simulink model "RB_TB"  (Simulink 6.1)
settings: Solver=ode3  SolverMode=SingleTasking  StartTime=0  StopTime=1000  FixedStep=0.05  RelTol=1e-3
libraries: simulink x2
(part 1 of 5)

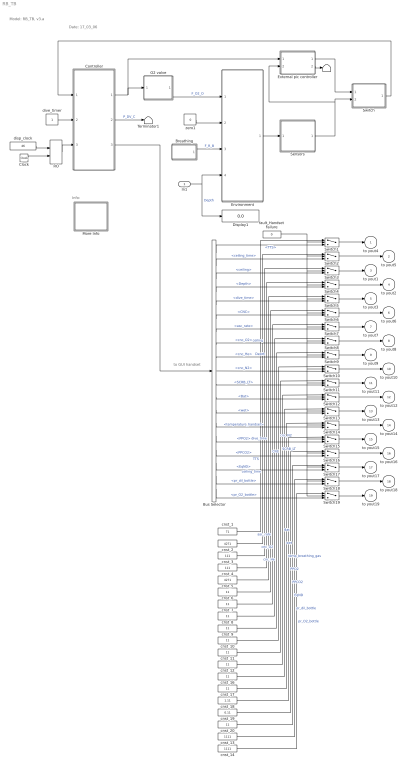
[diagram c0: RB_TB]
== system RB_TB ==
  note: Model: RB_TB, v3.a
  note: Date: 17_03_06
  note: to GUI handset
  note: Info:
  In1 : Inport  Port=1  LatchInput=off
  Breathing : Subsystem
  Bus Selector : BusSelector  DialogController=Simulink.DDGSource_Bus  OutputSignals=TTS,ceiling_time,ceiling,Depth,dive_time,CNC,asc_rate,cnc_O2,cnc_He,cnc_N2,SCRB_LT,Bat,wet,temperature_handset,PPO2,PPCO2,EqND,pr_dil_bottle,pr_O2_bottle
  Clock : Clock
  Controller : Subsystem
  Display1 : Display
  Environment : Subsystem
  External pic controller : Subsystem
  More Info : Subsystem
  O2 valve : Subsystem
  RO : RelationalOperator  Operator===  LogicOutDataTypeMode=Boolean
  Sensors : Subsystem
  Switch : Subsystem
  Switch{1..19} (19 alike) : Switch  Threshold=0.5
  T : Terminator
  Terminator1 : Terminator
  cnst_1 : Constant  Value=71
  cnst_{6..12,16..17,20} (10 alike) : Constant  Value=11
  cnst_13 : Constant  Value=1111
  cnst_14 : Constant  Value=1111
  cnst_18 : Constant  Value=1.11
  cnst_19 : Constant  Value=0.11
  cnst_2 : Constant  Value=4271
  cnst_3 : Constant  Value=111
  cnst_4 : Constant  Value=111
  cnst_5 : Constant  Value=4271
  disp_clock : Constant  Value=46
  dive_timer : Constant
  fault_Handset Failure : Constant  Value=0
  zero1 : Constant  Value=0
  to yout4 : Outport
  to yout5 : Outport  Port=2
  to yout1 : Outport  Port=3
  to yout2 : Outport  Port=4
  to yout3 : Outport  Port=5
  to yout6 : Outport  Port=6
  to yout7 : Outport  Port=7
  to yout8 : Outport  Port=8
  to yout9 : Outport  Port=9
  to yout10 : Outport  Port=10
  to yout11 : Outport  Port=11
  to yout12 : Outport  Port=12
  to yout13 : Outport  Port=13
  to yout14 : Outport  Port=14
  to yout15 : Outport  Port=15
  to yout16 : Outport  Port=16
  to yout17 : Outport  Port=17
  to yout18 : Outport  Port=18
  to yout19 : Outport  Port=19
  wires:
  Controller/1(O2 control) -> O2 valve/1(IN), External pic controller/1(valve_in)
  Breathing/1(Metabolic) -> Environment/3(Metablic)  "F_R_B"
  Environment/1(bus) -> Sensors/1(In)
  disp_clock/1 -> RO/1
  Clock/1 -> RO/2
  RO/1 -> Controller/3(disp_clock)
  External pic controller/1(sensor_out) -> Switch/1(In1)
  Sensors/1(Out) -> Switch/2(In2), External pic controller/2(sensor_in)
  Switch/1(Out) -> Controller/1(InBus)
  Controller/2(Dil valve) -> Terminator1/1  "P_DV_C"
  zero1/1 -> Environment/2(Dil valve)
  O2 valve/1(Orf_size) -> Environment/1(Orf_size)  "F_O2_O"
  dive_timer/1 -> Controller/2(dive_timer)
  cnst_1/1 -> Switch1/1  "TTS"
  cnst_2/1 -> Switch2/1  "ceiling_time"
  cnst_3/1 -> Switch3/1  "ceiling"
  cnst_4/1 -> Switch4/1  "Depth"
  cnst_5/1 -> Switch5/1  "dive_time"
  cnst_6/1 -> Switch6/1  "CNC"
  cnst_7/1 -> Switch7/1  "asc_rate"
  cnst_8/1 -> Switch8/1  "cnc_O2"
  cnst_9/1 -> Switch9/1  "cnc_He"
  cnst_10/1 -> Switch10/1  "cnc_N2"
  cnst_11/1 -> Switch11/1  "SCRB_LT"
  cnst_12/1 -> Switch12/1  "Bat"
  cnst_16/1 -> Switch13/1  "wet"
  cnst_17/1 -> Switch14/1  "temp_breathing_gas"
  cnst_18/1 -> Switch15/1  "PPO2"
  cnst_19/1 -> Switch16/1  "PPCO2"
  cnst_20/1 -> Switch17/1  "EqND"
  cnst_13/1 -> Switch18/1  "pr_dil_bottle"
  cnst_14/1 -> Switch19/1  "pr_O2_bottle"
  Controller/3(bus) -> Bus Selector/1
  Bus Selector/1 -> Switch1/3  "<TTS>"
  Bus Selector/2 -> Switch2/3  "<ceiling_time>"
  Bus Selector/3 -> Switch3/3  "<ceiling>"
  Bus Selector/4 -> Switch4/3  "<Depth>"
  Bus Selector/5 -> Switch5/3  "<dive_time>"
  Bus Selector/6 -> Switch6/3  "<CNC>"
  Bus Selector/7 -> Switch7/3  "<asc_rate>"
  Bus Selector/8 -> Switch8/3  "<cnc_O2>"
  Bus Selector/9 -> Switch9/3  "<cnc_He>"
  Bus Selector/10 -> Switch10/3  "<cnc_N2>"
  Bus Selector/11 -> Switch11/3  "<SCRB_LT>"
  Bus Selector/12 -> Switch12/3  "<Bat>"
  Bus Selector/13 -> Switch13/3  "<wet>"
  Bus Selector/14 -> Switch14/3  "<temperature_handset>"
  Bus Selector/15 -> Switch15/3  "<PPO2>"
  Bus Selector/16 -> Switch16/3  "<PPCO2>"
  Bus Selector/17 -> Switch17/3  "<EqND>"
  Bus Selector/18 -> Switch18/3  "<pr_dil_bottle>"
  Bus Selector/19 -> Switch19/3  "<pr_O2_bottle>"
  Switch19/1 -> to yout19/1
  Switch18/1 -> to yout18/1
  Switch17/1 -> to yout17/1
  Switch16/1 -> to yout16/1
  Switch15/1 -> to yout15/1
  Switch14/1 -> to yout14/1
  Switch13/1 -> to yout13/1
  Switch12/1 -> to yout12/1
  Switch11/1 -> to yout11/1
  Switch10/1 -> to yout10/1
  Switch9/1 -> to yout9/1
  Switch8/1 -> to yout8/1
  Switch7/1 -> to yout7/1
  Switch6/1 -> to yout6/1
  Switch5/1 -> to yout3/1
  Switch4/1 -> to yout2/1
  Switch3/1 -> to yout1/1
  Switch2/1 -> to yout5/1
  Switch1/1 -> to yout4/1
  fault_Handset Failure/1 -> Switch18/2, Switch19/2, Switch17/2, Switch16/2, Switch15/2, Switch14/2, Switch13/2, Switch12/2, Switch11/2, Switch10/2, Switch9/2, Switch8/2, Switch7/2, Switch6/2, Switch5/2, Switch4/2, Switch3/2, Switch2/2, Switch1/2
  In1/1 -> Display1/1, Environment/4(Depth)  "Depth"
  External pic controller/2(valve_out) -> T/1

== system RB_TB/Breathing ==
  note: Model: RB_TB/Breathing
  methabolic profile 1l/s : DiscretePulseGenerator  PulseType=Time based  Amplitude=2.5  PulseWidth=40
  product1 : Product
  rate_metabolic : Constant  Value=1.88
  scale : Gain  Gain=1/60
  Metabolic : Outport
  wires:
  methabolic profile 1l/s/1 -> product1/2
  product1/1 -> Metabolic/1  "l/s"
  scale/1 -> product1/1  "l/s"
  rate_metabolic/1 -> scale/1  "l/min"

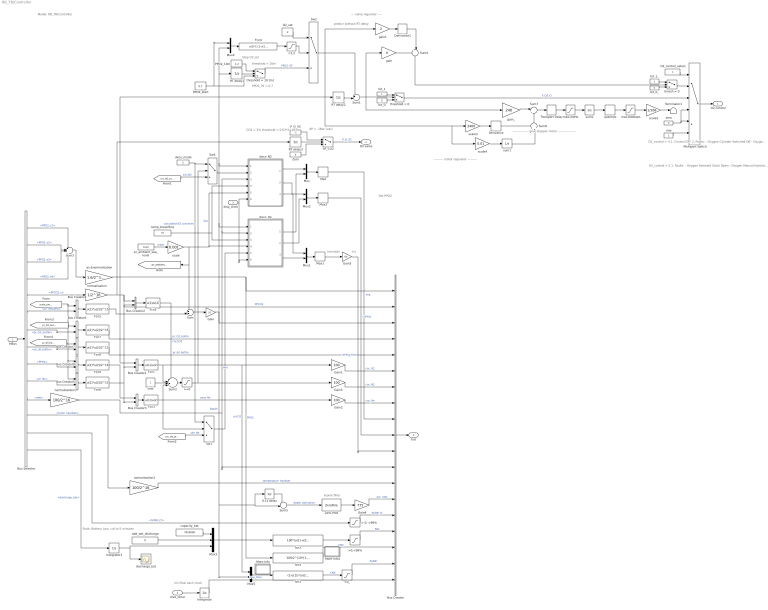
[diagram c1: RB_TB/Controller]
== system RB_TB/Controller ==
  note: Model: RB_TB/Controller
  note: dP = -1Bar (var)
  note: PPO2_ini = 0.7
  note: threshold = 10m
  note: CO2 = 3% threshold = 0.03*2^16
  note: (minute)
  note: (s)
  note: Step O2 set
  note: ini=final each clock
  note: Fault: Battery Low, cut to 5 minutes
  note: predicr without RT delay
  note: O2_control = 4 1. Control OFF 2. Faults: - Oxygen Cylinder Switched Off - Oxygen First Stage Failure - Oxygen Solenoid Stuck Closed
  note: O2_control = 5 1. Faults: - Oxygen Solenoid Stuck Open - Oxygen Manual Injector Failure
  note: 6-pole filter
  note: --------------- gear stepper motor -----------------
  note: Set PPO2
  note: --------- motor regulator ---------
  note: --- valve regulator ----
  InBus : Inport  Port=1  LatchInput=off
  dive_timer : Inport  Port=2  LatchInput=off
  disp_clock : Inport  Port=3  LatchInput=off
  0.1s delay : UnitDelay  SampleTime=0.1
  <1.2 : Saturate  UpperLimit=1.2  LowerLimit=0
  "> 0, <99%" : Saturate  UpperLimit=99  LowerLimit=0
  >0,<99% : Saturate  UpperLimit=99  LowerLimit=0
  >0_ : Saturate  UpperLimit=inf  LowerLimit=0
  >=0 : Saturate  UpperLimit=inf  LowerLimit=0
  Bus Creator : BusCreator  DialogController=Simulink.DDGSource_Bus  Inputs=19
  Bus Creator{1..8} (8 alike) : BusCreator  DialogController=Simulink.DDGSource_Bus  Inputs=2
  Bus Selector : BusSelector  DialogController=Simulink.DDGSource_Bus  OutputSignals=PPO2_s1,PPO2_s2,PPO2_s3,PPO2_s4,PPCO2_s,pr_ambient,pr_O2_bottle,pr_dil_bottle,PPHe,pr_BL,wet,temp_handset,SCRB_LT,discharge_bat
  Derivative : Derivative
  Derivative1 : Derivative
  Fcn1 : Fcn  Expr=u(1)/u(2)
  Fcn2 : Fcn  Expr=u(1)/u(2)
  Fcn3 : Fcn  Expr=u(1)/u(2)
  Fcn4 : Fcn  Expr=u(2)*(1.2-u(1))/10+u(1)
  Fcn{5..8} (4 alike) : Fcn  Expr=u(1)*u(2)/2^15
  Fcn9 : Fcn  Expr=u(1)*u(2)/2^16
  Gain : Gain  Gain=10
  Gain1 : Gain  Gain=100
  Gain2 : Gain  Gain=100
  Gain3 : Gain  Gain=60
  Gain4 : Gain  Gain=775
  Gain5 : Gain  Gain=100
  Integrator : Integrator
  Integrator1 : Integrator
  Max : MinMax  Function=max
  Max1 : MinMax  Function=max
  Max2 : MinMax  Function=max
  More Info : Subsystem
  More Info1 : Subsystem
  Multiport Switch : MultiPortSwitch  Inputs=5
  Mux{,1..2,4..5} (5 alike) : Mux  Inputs=2
  Mux3 : Mux  Inputs=3
  O2_control_select : Constant
  O2_set : Constant  Value=2
  PPO2_10m : Constant  Value=1.2
  PPO2_start : Constant  Value=0.7
  P_D_VC : Constant  Value=-1
  RT delay1 : UnitDelay  SampleTime=0.1
  RT delay2 : UnitDelay  SampleTime=0.1
  RT delay3 : UnitDelay  SampleTime=0.1
  SP_CO2 : Switch  Threshold=0.03
  Sum : Sum  Inputs=-+|
  Sum1 : Sum  Inputs=+-|
  Sum2 : Sum  Inputs=--+-|
  Sum3 : Sum  Inputs=++++
  Sum4 : Sum  Orientation=down  Inputs=+-|
  Sum5 : Sum  Inputs=-+|
  Sum7 : Sum  Inputs=|+-
  Sum8 : Sum  Orientation=up  Inputs=++|
  Sw1 : MultiPortSwitch  Inputs=2
  Sw2 : MultiPortSwitch  Inputs=2
  Sw4 : MultiPortSwitch  Inputs=2
  Terminator1 : Terminator
  Transport Delay : TransportDelay  DelayTime=0.01
  Zero : Constant  Value=0
  Zero-Pole : ZeroPole  Zeros=[0]  Poles=[-1 -1 -1 -1 -1 -1]
  add_bat_discharge : Constant  Value=0
  av.&normalisation : Gain  Gain=1.6/2^16/4
  bit_0 : Constant  Value=0
  bit_0_ : Constant  Value=0
  bit_1 : Constant
  bit_1_ : Constant
  capacity_bat : Constant  Value=7920000
  cnst : Constant
  deco_He : Subsystem
  deco_N2 : Subsystem
  deco_mode : Constant  Value=2
  discharge_bat : Scope
  fcn2 : Fcn  Expr=100*(u(1)-u(2)-u(3))/u(1)
  fcn3 : Fcn  Expr=(1-u(1))*(u(2)+10)/0.79-10
  fcn4 : Fcn  Expr=100/2^(10*(1.6 - u(1)))
  gain : Gain
  gain1 : Gain  Gain=2
  gain_ : Gain  Gain=240
  max100Hz : Saturate  UpperLimit=100  LowerLimit=-100
  max168steps : Saturate  UpperLimit=168  LowerLimit=0
  normalisation : Gain  Gain=1/2^16
  normalisation1 : Gain  Gain=100/2^16
  normalisation2 : Gain  Gain=100/2^16
  one : Constant
  pr_ambient_sea_level : Constant  Value=1010
  quantize : Quantizer  QuantizationInterval=1
  scale : Gain  Gain=0.001
  scale2 : Gain  Gain=1/168
  scale3 : Gain  Gain=3400
  scale4 : Gain  Gain=0.01
  sum1 : Integrator
  sum2 : Integrator
  temp_breathing : Constant  Value=33
  thresh = 0 : Switch  Criteria=u2 > Threshold
  threshold = 0 : Switch  Criteria=u2 > Threshold
  threshold = 10 [m] : Switch  Threshold=10
  zero : Constant  Value=0
  O2 control : Outport
  Dil valve : Outport  Port=2
  bus : Outport  Port=3
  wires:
  RT delay2/1 -> Sum1/2
  RT delay1/1 -> threshold = 10 [m]/2
  PPO2_start/1 -> threshold = 10 [m]/3, Mux4/1
  PPO2_10m/1 -> threshold = 10 [m]/1
  bit_1/1 -> threshold = 0/1
  bit_0/1 -> threshold = 0/3
  temp_breathing/1 -> deco_N2/4(Temp_air), deco_He/3(Temp_air)
  deco_N2/1(TTS_N2) -> Mux/1
  deco_He/1(TTS_He) -> Mux/2
  Mux/1 -> Max/1
  Mux1/1 -> Max1/1
  deco_He/3(ceiling_time_He) -> Mux1/2
  deco_N2/3(ceiling_time_N2) -> Mux1/1
  Mux2/1 -> Max2/1
  deco_N2/2(ceiling_N2) -> Mux2/1
  deco_He/2(ceiling_He) -> Mux2/2
  Max/1 -> Bus Creator/9  "TTS"
  Max2/1 -> Bus Creator/10  "ceiling"
  pr_ambient_sea_level/1 -> scale/1  "mbar"
  Bus Creator/1 -> bus/1
  InBus/1 -> Bus Selector/1
  Bus Selector/3 -> Sum3/3  "<PPO2_s3>"
  Bus Selector/4 -> Sum3/4  "<PPO2_s4>"
  av.&normalisation/1 -> Bus Creator1/1, Bus Creator/1, fcn4/1, RT delay2/1, gain1/1, scale3/1, scale4/1  "PPO2"
  normalisation/1 -> RT delay3/1, Bus Creator2/1, Bus Creator/2  "PPCO2"
  Sum/1 -> Gain/1
  Gain/1 -> Bus Creator/3, deco_He/1(depth), deco_N2/1(depth), RT delay1/1, Mux4/2, Mux5/2, 0.1s delay/1, Sum5/2  "Depth"
  Gain5/1 -> Bus Creator/7  "cnc_N2"
  Fcn3/1 -> Sum2/4, Sw1/2, Gain2/1  "sens He"
  disp_clock/1 -> deco_N2/6(disp_clock), deco_He/6(disp_clock)
  Integrator/1 -> Bus Creator/19  "dive_time"
  >0,<99%/1 -> Bus Creator/16  "Bat"
  >0_/1 -> Bus Creator/18  "EqND"
  RT delay3/1 -> SP_CO2/2
  P_D_VC/1 -> SP_CO2/1
  SP_CO2/1 -> Dil valve/1  "P_D_VC"
  Zero/1 -> SP_CO2/3
  Bus Selector/5 -> normalisation/1  "<PPCO2_s>"
  scale/1 -> deco_He/4(P_amb_sea_level), deco_N2/5(P_amb_sea_level), Sum/1, [pr_ambient_sea_level]  "bar"
  Max1/1 -> Gain3/1
  Gain3/1 -> Bus Creator/11  "ceiling_time"
  Mux3/1 -> fcn2/1
  fcn2/1 -> >0,<99%/1
  Fcn1/1 -> Sum2/2, Gain1/1, Mux5/1  "cncO2"
  Gain1/1 -> Bus Creator/6  "cnc_O2"
  Gain2/1 -> Bus Creator/8  "cnc_He"
  Bus Creator2/1 -> Fcn2/1
  cnst/1 -> Sum2/3
  Fcn2/1 -> Sum2/1  "cncCO2"
  deco_mode/1 -> Sw4/1, Sw1/1
  [cnc_N2_presize] -> Sw4/3  "sim N2"
  [cnc_He_presize] -> Sw1/3  "sim He"
  Sw4/1 -> deco_N2/2(cnc_N2)
  Sw1/1 -> deco_He/5(cnc_He)
  O2_set/1 -> Sw2/1
  threshold = 10 [m]/1 -> Sw2/3  "PPO2_SP"
  Sw2/1 -> Sum1/1
  Mux4/1 -> Fcn4/1
  <1.2/1 -> Sw2/2
  Fcn4/1 -> <1.2/1
  Mux5/1 -> fcn3/1
  fcn3/1 -> >0_/1  "CNS"
  fcn4/1 -> Bus Creator/17  "CNC"
  dive_timer/1 -> Integrator/1
  capacity_bat/1 -> Mux3/1
  add_bat_discharge/1 -> Mux3/2
  Integrator1/1 -> discharge_bat/1, Mux3/3
  Bus Selector/2 -> Sum3/2  "<PPO2_s2>"
  Bus Selector/1 -> Sum3/1  "<PPO2_s1>"
  Sum3/1 -> av.&normalisation/1
  Sum1/1 -> gain/1, threshold = 0/2, gain_/1
  gain1/1 -> Derivative1/1
  O2_control_select/1 -> Multiport Switch/1
  Multiport Switch/1 -> O2 control/1
  bit_1_/1 -> thresh = 0/1
  bit_0_/1 -> thresh = 0/3
  Sum4/1 -> thresh = 0/2
  thresh = 0/1 -> Multiport Switch/2
  threshold = 0/1 -> Multiport Switch/3  "F_O2_O"
  "> 0, <99%"/1 -> Bus Creator/15  "SCRB_LT"
  Bus Selector/14 -> Integrator1/1  "<discharge_bat>"
  Bus Selector/13 -> "> 0, <99%"/1  "<SCRB_LT>"
  Bus Selector/11 -> normalisation1/1  "<wet>"
  normalisation1/1 -> deco_He/2(Wet), deco_N2/3(Wet), Bus Creator/12  "wet"
  Bus Selector/12 -> normalisation2/1  "<temp_handset>"
  normalisation2/1 -> Bus Creator/13  "temperature_handset"
  [scale_pressure] -> Bus Creator4/1, Bus Creator5/1, Bus Creator8/1
  Bus Selector/6 -> Bus Creator4/2  "<pr_ambient>"
  Bus Creator4/1 -> Fcn5/1
  Fcn5/1 -> Sum/2
  Sum2/1 -> >=0/1
  >=0/1 -> Gain5/1, Sw4/2  "calculated N2 concentration"
  one/1 -> Multiport Switch/6
  zero/1 -> Multiport Switch/5, Multiport Switch/4
  Bus Creator3/1 -> Fcn3/1
  Bus Creator1/1 -> Fcn1/1
  Bus Creator5/1 -> Fcn6/1
  Bus Selector/10 -> Bus Creator5/2  "<pr_BL>"
  Fcn6/1 -> Bus Creator3/2, Bus Creator1/2, Bus Creator2/2
  Sum5/1 -> Zero-Pole/1  "depth_derivative"
  0.1s delay/1 -> Sum5/1
  Zero-Pole/1 -> Gain4/1
  Gain4/1 -> Bus Creator/14  "asc_rate"
  Bus Selector/7 -> Bus Creator6/2  "<pr_O2_bottle>"
  Fcn7/1 -> Bus Creator/4  "pr_O2_bottle"
  Bus Creator6/1 -> Fcn7/1
  [pr_O2_bottle_ini] -> Bus Creator6/1
  Bus Creator7/1 -> Fcn8/1
  Fcn8/1 -> Bus Creator/5  "pr_dil_bottle"
  Bus Selector/8 -> Bus Creator7/2  "<pr_dil_bottle>"
  [pr_dil_bottle_ini] -> Bus Creator7/1
  Bus Creator8/1 -> Fcn9/1
  Bus Selector/9 -> Bus Creator8/2  "<PPHe>"
  Fcn9/1 -> Bus Creator3/1
  max168steps/1 -> scale2/1
  quantize/1 -> max168steps/1
  sum2/1 -> quantize/1
  max100Hz/1 -> sum2/1
  Transport Delay/1 -> max100Hz/1
  Sum7/1 -> Transport Delay/1
  scale3/1 -> Derivative/1
  scale4/1 -> sum1/1
  gain_/1 -> Sum7/1
  Derivative/1 -> Sum8/1
  Sum8/1 -> Sum7/2
  gain/1 -> Sum4/1
  Derivative1/1 -> Sum4/2
  sum1/1 -> Sum8/2
  scale2/1 -> Terminator1/1

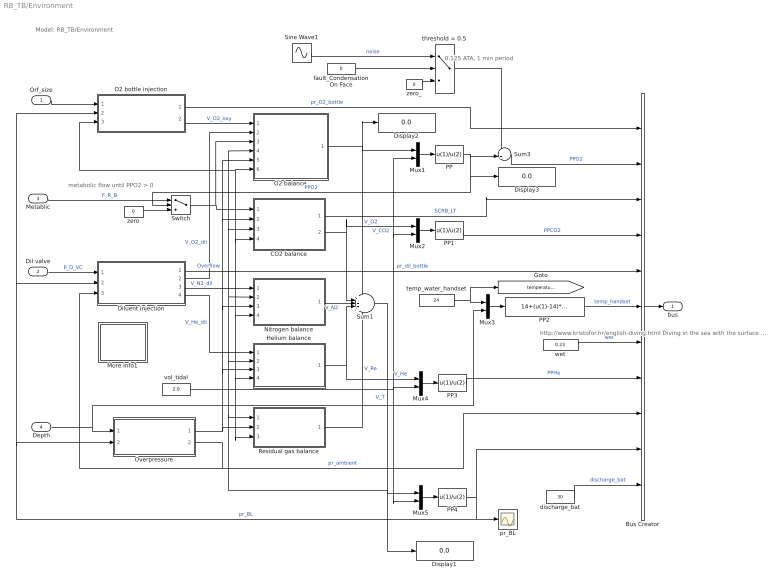
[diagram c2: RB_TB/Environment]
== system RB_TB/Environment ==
  note: Model: RB_TB/Environment
  note: metabolic flow until PPO2 > 0
  note: 0.125 ATA, 1 min period
  note: http://www.kristofor.hr/english-diving.html Diving in the sea with the surface sea temperature 9 - 12 deg.C in winter, 24 - 28 degC in summer, On 20 m sea depth temperature is permanent, around 14 deg.C
  Orf_size : Inport  Port=1  LatchInput=off
  Dil valve : Inport  Port=2  LatchInput=off
  Metablic : Inport  Port=3  LatchInput=off
  Depth : Inport  Port=4  LatchInput=off
  Bus Creator : BusCreator  DialogController=Simulink.DDGSource_Bus  Inputs=11
  CO2 balance : Subsystem
  Diluent injection : Subsystem
  Display1 : Display
  Display2 : Display
  Display3 : Display
  Helium balance : Subsystem
  More Info1 : Subsystem
  Mux{1..5} (5 alike) : Mux  Inputs=2
  Nitrogen balance : Subsystem
  O2 balance : Subsystem
  O2 bottle injection : Subsystem
  Overpressure : Subsystem
  PP{,1,3..4} (4 alike) : Fcn  Tag=ee  Priority=306454640  Expr=u(1)/u(2)
  PP2 : Fcn  Tag=ee  Priority=306454640  Expr=14+(u(1)-14)*exp(-u(2)/7)
  Residual gas balance : Subsystem
  Sine Wave1 : Sin  Amplitude=0.125  Frequency=pi/30  SampleTime=0
  Sum1 : Sum  Inputs=+++++
  Sum3 : Sum  Inputs=++|
  Switch : Switch  Criteria=u2 > Threshold
  discharge_bat : Constant  Value=30
  fault_Condensation On Face : Constant  Value=0
  pr_BL : Scope
  temp_water_handset : Constant  Value=24
  threshold = 0.5 : Switch  Criteria=u2 > Threshold  Threshold=0.5
  vol_tidal : Constant  Value=2.0
  wet : Constant  Value=0.23
  zero : Constant  Value=0
  zero_ : Constant  Value=0
  bus : Outport
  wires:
  Diluent injection/3(N2) -> Nitrogen balance/1(V_N2_dil)  "V_N2_dil"
  Diluent injection/2(O2) -> O2 balance/2(V_O2_dil)  "V_O2_dil"
  O2 balance/1(O2 inside) -> Sum1/1, Mux1/1, Display2/1  "V_O2"
  Overpressure/1(Overflow) -> CO2 balance/2(Overflow), O2 balance/5(Overflow), Nitrogen balance/3(Overflow), Helium balance/3(Overflow), Residual gas balance/2(Overflow)  "Overflow"
  Sum1/1 -> Mux5/1, Helium balance/2(gas_total), Nitrogen balance/2(gas_total), CO2 balance/3(gas_total), O2 balance/4(gas_total), Residual gas balance/1(gas_total), Display1/1  "V_T"
  Nitrogen balance/1(N2 inside) -> Sum1/3  "V_N2"
  CO2 balance/2(CO2) -> Sum1/2, Mux2/1  "V_CO2"
  Dil valve/1 -> Diluent injection/1(Valve_ON/OFF)  "P_D_VC"
  Helium balance/1(He inside) -> Mux4/1, Sum1/4  "V_He"
  Diluent injection/4(He) -> Helium balance/1(V_He_dil)  "V_He_dil"
  Residual gas balance/1(Re inside) -> Sum1/5  "V_Re"
  PP/1 -> Sum3/2, Switch/2, Display3/1  "PPO2"
  Bus Creator/1 -> bus/1
  PP1/1 -> Bus Creator/4  "PPCO2"
  PP3/1 -> Bus Creator/8  "PPHe"
  vol_tidal/1 -> Helium balance/4(vol_tidal), Nitrogen balance/4(vol_tidal), CO2 balance/4(vol_tidal), O2 balance/6(vol_tidal), O2 bottle injection/3(vol_tidal), Residual gas balance/3(vol_tidal), Mux4/2, Mux2/2, Mux1/2, Mux5/2
  Mux1/1 -> PP/1
  Mux2/1 -> PP1/1
  Mux4/1 -> PP3/1
  Orf_size/1 -> O2 bottle injection/1(Orf_size)
  O2 bottle injection/2(V_O2_oxygen_bottle) -> O2 balance/1(V_O2_oxy)  "V_O2_oxy"
  O2 bottle injection/1(pr_O2_bottle) -> Bus Creator/1  "pr_O2_bottle"
  wet/1 -> Bus Creator/7  "wet"
  Overpressure/2(pr_ambient) -> Bus Creator/9, Diluent injection/3(pr_ambient)  "pr_ambient"
  Diluent injection/1(pr_dil_bottle) -> Bus Creator/5  "pr_dil_bottle"
  Mux5/1 -> PP4/1
  PP4/1 -> Bus Creator/10, pr_BL/1, O2 bottle injection/2(pr_BL), Diluent injection/2(pr_BL), Overpressure/2(pr_BL)  "pr_BL"
  Depth/1 -> Overpressure/1(Depth), Mux3/2
  Switch/1 -> CO2 balance/1(Metabolic), O2 balance/3(Metabolic)
  Metablic/1 -> Switch/1  "F_R_B"
  zero/1 -> Switch/3
  CO2 balance/1(SCRB) -> Bus Creator/3  "SCRB_LT"
  discharge_bat/1 -> Bus Creator/11  "discharge_bat"
  fault_Condensation On Face/1 -> threshold = 0.5/2
  Sine Wave1/1 -> threshold = 0.5/1  "noise"
  zero_/1 -> threshold = 0.5/3
  Sum3/1 -> Bus Creator/2  "PPO2"
  threshold = 0.5/1 -> Sum3/1
  temp_water_handset/1 -> Mux3/1, [temperature_sea_level]
  Mux3/1 -> PP2/1
  PP2/1 -> Bus Creator/6  "temp_handset"

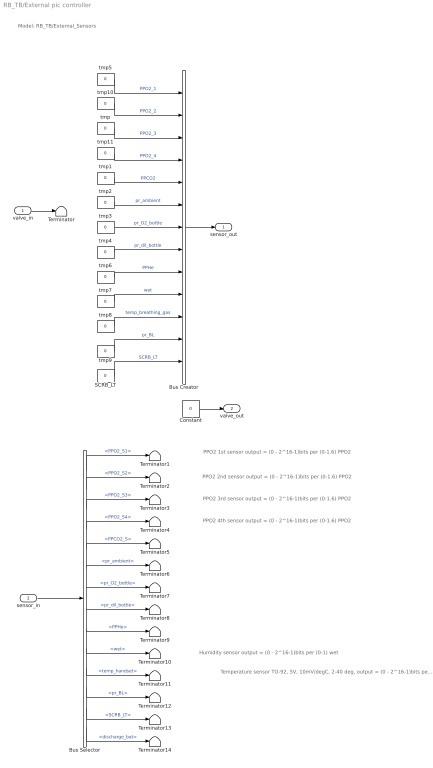
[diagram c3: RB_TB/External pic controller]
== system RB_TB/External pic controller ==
  note: Model: RB_TB/External_Sensors
  note: Humidity sensor output = (0 - 2^16-1)bits per (0-1) wet
  note: PPO2 1st sensor output = (0 - 2^16-1)bits per (0-1.6) PPO2
  note: PPO2 2nd sensor output = (0 - 2^16-1)bits per (0-1.6) PPO2
  note: PPO2 3rd sensor output = (0 - 2^16-1)bits per (0-1.6) PPO2
  note: PPO2 4th sensor output = (0 - 2^16-1)bits per (0-1.6) PPO2
  note: Temperature sensor TO-92, 5V, 10mV/degC, 2-40 deg, output = (0 - 2^16-1)bits per (0-1) wet
  valve_in : Inport  Port=1  LatchInput=off
  sensor_in : Inport  Port=2  LatchInput=off
  Bus Creator : BusCreator  DialogController=Simulink.DDGSource_Bus  Inputs=13
  Bus Selector : BusSelector  DialogController=Simulink.DDGSource_Bus  OutputSignals=PPO2_S1,PPO2_S2,PPO2_S3,PPO2_S4,PPCO2_S,pr_ambient,pr_O2_bottle,pr_dil_bottle,PPHe,wet,temp_handset,pr_BL,SCRB_LT,discharge_bat
  Constant : Constant  Value=0
  SCRB_LT : Constant  Value=0
  Terminator{,1..14} (15 alike) : Terminator
  tmp{,1..11} (12 alike) : Constant  Value=0
  sensor_out : Outport
  valve_out : Outport  Port=2
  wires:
  tmp7/1 -> Bus Creator/10  "wet"
  tmp8/1 -> Bus Creator/11  "temp_breathing_gas"
  tmp6/1 -> Bus Creator/9  "PPHe"
  tmp4/1 -> Bus Creator/8  "pr_dil_bottle"
  tmp3/1 -> Bus Creator/7  "pr_O2_bottle"
  tmp2/1 -> Bus Creator/6  "pr_ambient"
  tmp1/1 -> Bus Creator/5  "PPCO2"
  Bus Creator/1 -> sensor_out/1
  tmp/1 -> Bus Creator/3  "PPO2_3"
  valve_in/1 -> Terminator/1
  tmp9/1 -> Bus Creator/12  "pr_BL"
  SCRB_LT/1 -> Bus Creator/13  "SCRB_LT"
  tmp5/1 -> Bus Creator/1  "PPO2_1"
  tmp10/1 -> Bus Creator/2  "PPO2_2"
  sensor_in/1 -> Bus Selector/1
  tmp11/1 -> Bus Creator/4  "PPO2_4"
  Bus Selector/1 -> Terminator1/1  "<PPO2_S1>"
  Bus Selector/2 -> Terminator2/1  "<PPO2_S2>"
  Bus Selector/3 -> Terminator3/1  "<PPO2_S3>"
  Bus Selector/4 -> Terminator4/1  "<PPO2_S4>"
  Bus Selector/5 -> Terminator5/1  "<PPCO2_S>"
  Bus Selector/9 -> Terminator9/1  "<PPHe>"
  Bus Selector/6 -> Terminator6/1  "<pr_ambient>"
  Bus Selector/7 -> Terminator7/1  "<pr_O2_bottle>"
  Bus Selector/8 -> Terminator8/1  "<pr_dil_bottle>"
  Bus Selector/10 -> Terminator10/1  "<wet>"
  Bus Selector/11 -> Terminator11/1  "<temp_handset>"
  Bus Selector/12 -> Terminator12/1  "<pr_BL>"
  Bus Selector/13 -> Terminator13/1  "<SCRB_LT>"
  Bus Selector/14 -> Terminator14/1  "<discharge_bat>"
  Constant/1 -> valve_out/1

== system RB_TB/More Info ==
  note: The S-Function "depth_data" runs depth_data.m in real-time that calculates the current depth using the Depth table data. The Simulink subsytems are Valve controller and Breathing loop. Gas balance includes O2, CO2, N2, He and Reminder gas the O2 pressure reduction valve is not compensated to ambient pressure Controller includes: Bang-Bang O2 and CO2 control; calc of decompression The depth profile is profile.time = [time1, time2,..., timen], and profile.rate = [depth_ini, rate1, rate2,...raten ] 1b deco compartments for N2 and He are installed "a", "b" and Half-Time deco for H2 is updated tissue compartment of 1b deco for N2 and He are add the half_times of He are updated satuation of the PPO2 sensor is 1.6 round of the deco d_min is changed by ceil ceil of the deco ceiling time and asc_time is removed models of the SCRB, BAT, CNS and EqND parameters are installed 04_03_06 updated (limit is -inf) the non compensated O2 valve 05_03_06 compensated O2 valve is installed 08_03_06 flow through the orifice depends on its diameter and spring pressure 08_03_06 ADV and OVP value of 5-50mbar is defined via the GUI 09_03_06 Faults are attached 11_03_06 Range of Analog O2 set is (0.7 - 1.2 ATA)/(0-10m) 18_03_06 Nonlinear model of OPV and ADV valves are installed 18_03_06 Predictive Bang-Bang O2 valve control is installed 22_03_06 PPO2 and CO2 LED are installed 23_03_06 Sensors time constant and ADCs are installed 24_03_06 O2 and Dil manual injection is add 25_03_06 Sound of PAUSE and nonconnected modes is ON
  note: The run file is main_RB_TB.m
  note: Temporary actions: 1) The 0.1s delay of PPO2 sensor is removed
  note: This system models the Re-Breather Test Bench. It includs analogue and digital parts.
  note: PPCO2 controls is off

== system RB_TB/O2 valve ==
  note: Model: RB_TB/O2 valve
  IN : Inport  Port=1  LatchInput=off
  DAC 1bit : DataTypeConversion  OutDataTypeMode=double  ConvertRealWorld=Stored Integer (SI)  RndMeth=Nearest
  Orf_size : Outport
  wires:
  IN/1 -> DAC 1bit/1
  DAC 1bit/1 -> Orf_size/1

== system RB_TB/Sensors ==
  note: Model: RB_TB/Sensors
  note: Info:
  note: 5 mV corresponds to air PPO2 of 0.21 ATA
  In : Inport  Port=1  LatchInput=off
  5mV : Constant  Value=8580.1
  Bus Creator : BusCreator  DialogController=Simulink.DDGSource_Bus  Inputs=14
  Bus Selector : BusSelector  DialogController=Simulink.DDGSource_Bus  OutputSignals=PPO2,PPCO2,pr_ambient,pr_O2_bottle,pr_dil_bottle,PPHe,wet,temp_handset,pr_BL,SCRB_LT,discharge_bat
  Gain : Gain
  Gain1 : Gain
  Gain2 : Gain
  Humidity Sensor : Subsystem
  More Info : Subsystem
  PPCO2 sensor : Subsystem
  PPHe sensor : Subsystem
  PPO2 sensor : Subsystem
  Pressure_Br_Loop Sensor : Subsystem
  Pressure_O2_bottle_Sensor1 : Subsystem
  Pressure_ambient Sensor : Subsystem
  Pressure_dil_bottle_Sensor : Subsystem
  Temperature Sensor : Subsystem
  fault_Loose Connection to Sensor : Constant  Value=0
  fault_Single Cell Failure : Constant  Value=0
  fault_Two Cell Failure : Constant  Value=0
  thresh = 0.5 : Switch  Criteria=u2 > Threshold  Threshold=0.5
  threshold = 0.5 : Switch  Criteria=u2 > Threshold  Threshold=0.5
  threshold = 0.5_ : Switch  Criteria=u2 > Threshold  Threshold=0.5
  zero : Constant  Value=0
  Out : Outport
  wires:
  In/1 -> Bus Selector/1
  Bus Creator/1 -> Out/1
  Bus Selector/1 -> PPO2 sensor/1(PPO2)  "<PPO2>"
  Bus Selector/2 -> PPCO2 sensor/1(PPCO2)  "<PPCO2>"
  PPO2 sensor/1(PPO2_S) -> threshold = 0.5/3  "PPO2_S"
  PPCO2 sensor/1(PPCO2_S) -> Bus Creator/5  "PPCO2_S"
  Bus Selector/10 -> Bus Creator/13  "<SCRB_LT>"
  Bus Selector/11 -> Bus Creator/14  "<discharge_bat>"
  fault_Loose Connection to Sensor/1 -> threshold = 0.5/2
  threshold = 0.5/1 -> Gain/1, Gain1/1, Bus Creator/3, Gain2/1  "PPO2_S3"
  zero/1 -> threshold = 0.5/1
  fault_Single Cell Failure/1 -> threshold = 0.5_/2
  5mV/1 -> threshold = 0.5_/1, thresh = 0.5/1
  Gain1/1 -> threshold = 0.5_/3
  fault_Two Cell Failure/1 -> thresh = 0.5/2
  Gain/1 -> thresh = 0.5/3  "PPO2_S2"
  thresh = 0.5/1 -> Bus Creator/2  "PPO2_S2"
  threshold = 0.5_/1 -> Bus Creator/1  "PPO2_S1"
  Gain2/1 -> Bus Creator/4  "PPO2_S4"
  Bus Selector/7 -> Humidity Sensor/1(in)  "<wet>"
  Humidity Sensor/1(out) -> Bus Creator/10  "wet"
  Bus Selector/8 -> Temperature Sensor/1(in)  "<temp_handset>"
  Temperature Sensor/1(out) -> Bus Creator/11  "temp_handset"
  Bus Selector/3 -> Pressure_ambient Sensor/1(in)  "<pr_ambient>"
  Pressure_ambient Sensor/1(out) -> Bus Creator/6  "pr_ambient"
  Bus Selector/9 -> Pressure_Br_Loop Sensor/1(in)  "<pr_BL>"
  Pressure_Br_Loop Sensor/1(out) -> Bus Creator/12  "pr_BL"
  Bus Selector/5 -> Pressure_dil_bottle_Sensor/1(in)  "<pr_dil_bottle>"
  Pressure_dil_bottle_Sensor/1(out) -> Bus Creator/8  "pr_dil_bottle"
  Bus Selector/4 -> Pressure_O2_bottle_Sensor1/1(in)  "<pr_O2_bottle>"
  Pressure_O2_bottle_Sensor1/1(out) -> Bus Creator/7  "pr_O2_bottle"
  PPHe sensor/1(PPHe_S) -> Bus Creator/9  "PPHe"
  Bus Selector/6 -> PPHe sensor/1(PPHe)  "<PPHe>"

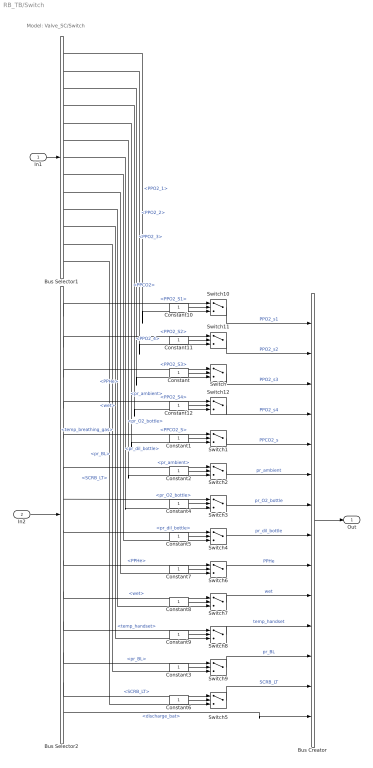
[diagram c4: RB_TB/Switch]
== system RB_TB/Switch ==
  note: Model: Valve_SC/Switch
  In1 : Inport  Port=1  LatchInput=off
  In2 : Inport  Port=2  LatchInput=off
  Bus Creator : BusCreator  DialogController=Simulink.DDGSource_Bus  Inputs=14
  Bus Selector1 : BusSelector  DialogController=Simulink.DDGSource_Bus  OutputSignals=PPO2_1,PPO2_2,PPO2_3,PPO2_4,PPCO2,pr_ambient,pr_O2_bottle,pr_dil_bottle,PPHe,wet,temp_breathing_gas,pr_BL,SCRB_LT
  Bus Selector2 : BusSelector  DialogController=Simulink.DDGSource_Bus  OutputSignals=PPO2_S1,PPO2_S2,PPO2_S3,PPO2_S4,PPCO2_S,pr_ambient,pr_O2_bottle,pr_dil_bottle,PPHe,wet,temp_handset,pr_BL,SCRB_LT,discharge_bat
  Constant{,1..12} (13 alike) : Constant
  Switch{,1..12} (13 alike) : Switch
  Out : Outport
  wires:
  Switch7/1 -> Bus Creator/10  "wet"
  Switch8/1 -> Bus Creator/11  "temp_handset"
  Switch6/1 -> Bus Creator/9  "PPHe"
  Switch4/1 -> Bus Creator/8  "pr_dil_bottle"
  Switch3/1 -> Bus Creator/7  "pr_O2_bottle"
  Switch2/1 -> Bus Creator/6  "pr_ambient"
  Switch1/1 -> Bus Creator/5  "PPCO2_s"
  Switch/1 -> Bus Creator/3  "PPO2_s3"
  Bus Creator/1 -> Out/1
  Bus Selector1/7 -> Switch3/3  "<pr_O2_bottle>"
  In1/1 -> Bus Selector1/1
  Bus Selector1/6 -> Switch2/3  "<pr_ambient>"
  Bus Selector1/5 -> Switch1/3  "<PPCO2>"
  Bus Selector1/4 -> Switch12/3  "<PPO2_4>"
  Bus Selector1/3 -> Switch/3  "<PPO2_3>"
  Bus Selector2/8 -> Switch4/1  "<pr_dil_bottle>"
  In2/1 -> Bus Selector2/1
  Bus Selector2/7 -> Switch3/1  "<pr_O2_bottle>"
  Bus Selector2/6 -> Switch2/1  "<pr_ambient>"
  Bus Selector2/5 -> Switch1/1  "<PPCO2_S>"
  Constant/1 -> Switch/2
  Constant1/1 -> Switch1/2
  Constant2/1 -> Switch2/2
  Constant4/1 -> Switch3/2
  Constant5/1 -> Switch4/2
  Constant7/1 -> Switch6/2
  Constant8/1 -> Switch7/2
  Constant9/1 -> Switch8/2
  Bus Selector2/12 -> Switch9/1  "<pr_BL>"
  Constant3/1 -> Switch9/2
  Switch9/1 -> Bus Creator/12  "pr_BL"
  Bus Selector2/9 -> Switch6/1  "<PPHe>"
  Bus Selector2/10 -> Switch7/1  "<wet>"
  Bus Selector2/11 -> Switch8/1  "<temp_handset>"
  Bus Selector1/8 -> Switch4/3  "<pr_dil_bottle>"
  Bus Selector1/9 -> Switch6/3  "<PPHe>"
  Bus Selector1/10 -> Switch7/3  "<wet>"
  Bus Selector1/11 -> Switch8/3  "<temp_breathing_gas>"
  Bus Selector2/13 -> Switch5/1  "<SCRB_LT>"
  Constant6/1 -> Switch5/2
  Switch5/1 -> Bus Creator/13  "SCRB_LT"
  Bus Selector1/12 -> Switch9/3  "<pr_BL>"
  Bus Selector2/14 -> Bus Creator/14  "<discharge_bat>"
  Constant10/1 -> Switch10/2
  Constant11/1 -> Switch11/2
  Switch11/1 -> Bus Creator/2  "PPO2_s2"
  Switch10/1 -> Bus Creator/1  "PPO2_s1"
  Bus Selector2/3 -> Switch/1  "<PPO2_S3>"
  Bus Selector2/2 -> Switch11/1  "<PPO2_S2>"
  Bus Selector2/1 -> Switch10/1  "<PPO2_S1>"
  Bus Selector1/2 -> Switch11/3  "<PPO2_2>"
  Bus Selector1/1 -> Switch10/3  "<PPO2_1>"
  Bus Selector2/4 -> Switch12/1  "<PPO2_S4>"
  Constant12/1 -> Switch12/2
  Switch12/1 -> Bus Creator/4  "PPO2_s4"
  Bus Selector1/13 -> Switch5/3  "<SCRB_LT>"

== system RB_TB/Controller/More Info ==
  note: END = (1-F02)/0.79*(Depth + 10) - 10 Where F02 is fraction of O2 in the gas: % divided by 100. For example, FO2 of air is 0.209 Imperial END = [(1 - FO2)*(Depth + 33)/0.79] - 33 END is the relative narcosis to air, that is, how narcotic the gas is compared to diving air. For example, if someone dives on Nitrox 32 (32% O2, 68% N2) then at 40m the narcosis is the same as on air to 33.05 meters
  note: E.N.D. (Equivalent Nitrogen Depth)

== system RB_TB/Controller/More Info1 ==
  note: CNS (Central Nervous System Toxicity)
  note: Ideally http://www.... The simple method, which we can use for now: A PPO2 of 1.6, has a CNS limit of 90 m?nutes. For every 0.1 above this, halve the time, every 0.1 below this, double the time. This gives the amount of the CNS used. For example, if I dive for 90 minutes at a PPO2 of 1.2, then I have used 1/16th of my CNS budget. Recovery of the CNS has a half life of 90 minutes. This means that in 90 minutes on air, then a 100% CNS penalty will reduce to 0.5 Most people assume that after 24 hours with no diving, the CNS clock is set to 0.

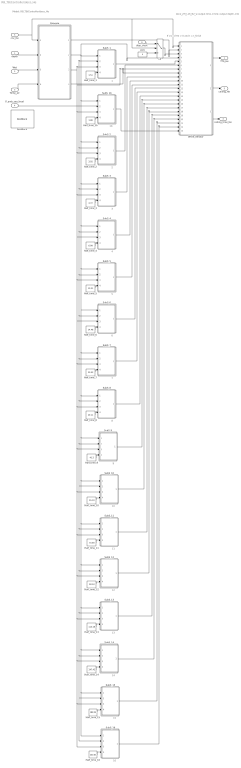
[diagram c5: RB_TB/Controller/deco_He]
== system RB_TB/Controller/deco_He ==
  note: 16
  note: 15
  note: 14
  note: 13
  note: 12
  note: 11
  note: 10
  note: 9
  note: 8
  note: 7
  note: 6
  note: 5
  note: 4
  note: 3
  note: 2
  note: 1
  note: deco_ZH_L16_N2_w output time, [min]; output depth, [m]
  note: Model: RB_TB/Controller/deco_He
  note: If cnc of He > 0 and t = t_finish
  note: 1b
  depth : Inport  Port=1  LatchInput=off
  Wet : Inport  Port=2  LatchInput=off
  Temp_air : Inport  Port=3  LatchInput=off
  P_amb_sea_level : Inport  Port=4  LatchInput=off
  cnc_He : Inport  Port=5  LatchInput=off
  disp_clock : Inport  Port=6  LatchInput=off
  >0 : Switch  Criteria=u2 > Threshold
  DocBlock : simulink/Model-Wide Utilities/DocBlock  DocumentType=Text
  Half_time_1 : Constant  Value=1.51
  Half_time_10 : Constant  Value=55.19
  Half_time_11 : Constant  Value=70.69
  Half_time_12 : Constant  Value=90.34
  Half_time_13 : Constant  Value=115.29
  Half_time_14 : Constant  Value=147.42
  Half_time_15 : Constant  Value=188.24
  Half_time_16 : Constant  Value=240.03
  Half_time_1b : Constant  Value=1.88
  Half_time_2 : Constant  Value=3.02
  Half_time_3 : Constant  Value=4.72
  Half_time_4 : Constant  Value=6.99
  Half_time_5 : Constant  Value=10.21
  Half_time_6 : Constant  Value=14.48
  Half_time_7 : Constant  Value=20.53
  Half_time_8 : Constant  Value=29.11
  Half_time_9 : Constant  Value=41.2
  Palveola : Subsystem
  SubS_1 : Subsystem
  SubS_10 : Subsystem
  SubS_11 : Subsystem
  SubS_12 : Subsystem
  SubS_13 : Subsystem
  SubS_14 : Subsystem
  SubS_15 : Subsystem
  SubS_16 : Subsystem
  SubS_1b : Subsystem
  SubS_2 : Subsystem
  SubS_3 : Subsystem
  SubS_4 : Subsystem
  SubS_5 : Subsystem
  SubS_6 : Subsystem
  SubS_7 : Subsystem
  SubS_8 : Subsystem
  SubS_9 : Subsystem
  While_Iterator : Subsystem  TreatAsAtomicUnit=on
  zero : Constant  Value=0
  TTS_He : Outport
  ceiling_He : Outport  Port=2
  ceiling_time_He : Outport  Port=3
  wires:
  Half_time_16/1 -> SubS_16/4(HT)
  Half_time_15/1 -> SubS_15/4(HT)
  Half_time_14/1 -> SubS_14/4(HT)
  Half_time_13/1 -> SubS_13/4(HT)
  Half_time_12/1 -> SubS_12/4(HT)
  Half_time_11/1 -> SubS_11/4(HT)
  Half_time_10/1 -> SubS_10/4(HT)
  Half_time_9/1 -> SubS_9/4(HT)
  Half_time_8/1 -> SubS_8/4(HT)
  Half_time_7/1 -> SubS_7/4(HT)
  Half_time_6/1 -> SubS_6/4(HT)
  Half_time_5/1 -> SubS_5/4(HT)
  Half_time_4/1 -> SubS_4/4(HT)
  Half_time_3/1 -> SubS_3/4(HT)
  Half_time_2/1 -> SubS_2/4(HT)
  Half_time_1/1 -> SubS_1/4(HT)
  SubS_16/1(bus) -> While_Iterator/22(In16)
  SubS_15/1(bus) -> While_Iterator/21(In15)
  SubS_14/1(bus) -> While_Iterator/20(In14)
  SubS_13/1(bus) -> While_Iterator/19(In13)
  SubS_12/1(bus) -> While_Iterator/18(In12)
  SubS_11/1(bus) -> While_Iterator/17(In11)
  SubS_10/1(bus) -> While_Iterator/16(In10)
  SubS_9/1(bus) -> While_Iterator/15(In9)
  SubS_8/1(bus) -> While_Iterator/14(In8)
  SubS_7/1(bus) -> While_Iterator/13(In7)
  SubS_6/1(bus) -> While_Iterator/12(In6)
  SubS_5/1(bus) -> While_Iterator/11(In5)
  SubS_4/1(bus) -> While_Iterator/10(In4)
  SubS_3/1(bus) -> While_Iterator/9(In3)
  Temp_air/1 -> Palveola/4(Temperature)
  Wet/1 -> Palveola/3(Humidity)
  While_Iterator/3(ceiling_time) -> ceiling_time_He/1
  While_Iterator/2(ceiling) -> ceiling_He/1
  While_Iterator/1(TTS) -> TTS_He/1
  Palveola/4(fnc_hum_temp) -> While_Iterator/8(fnc_hum_temp)
  Palveola/1(Psw) -> While_Iterator/2(Psw)
  SubS_1/1(bus) -> While_Iterator/5(In1)
  SubS_2/1(bus) -> While_Iterator/6(In2)
  cnc_He/1 -> Palveola/1(Gas concentration), >0/2, While_Iterator/1(cnc_He)
  depth/1 -> Palveola/2("depth, m ")
  Palveola/3(P_alv_INI) -> While_Iterator/7(Palv_INI), SubS_15/3(Palv_INI), SubS_16/3(Palv_INI), SubS_14/3(Palv_INI), SubS_13/3(Palv_INI), SubS_12/3(Palv_INI), SubS_11/3(Palv_INI), SubS_10/3(Palv_INI), SubS_9/3(Palv_INI), SubS_8/3(Palv_INI), SubS_7/3(Palv_INI), SubS_6/3(Palv_INI), SubS_5/3(Palv_INI), SubS_4/3(Palv_INI), SubS_3/3(Palv_INI), SubS_2/3(Palv_INI), SubS_1b/3(Palv_INI), SubS_1/3(Palv_INI)
  Palveola/2(Palv) -> While_Iterator/4(Palv), SubS_1/1(Palv), SubS_15/1(Palv), SubS_16/1(Palv), SubS_14/1(Palv), SubS_13/1(Palv), SubS_12/1(Palv), SubS_11/1(Palv), SubS_10/1(Palv), SubS_9/1(Palv), SubS_8/1(Palv), SubS_7/1(Palv), SubS_6/1(Palv), SubS_5/1(Palv), SubS_4/1(Palv), SubS_3/1(Palv), SubS_2/1(Palv), SubS_1b/1(Palv)
  P_amb_sea_level/1 -> SubS_1/2(Pamb_sea), SubS_15/2(Pamb_sea), SubS_16/2(Pamb_sea), SubS_14/2(Pamb_sea), SubS_13/2(Pamb_sea), SubS_12/2(Pamb_sea), SubS_11/2(Pamb_sea), SubS_10/2(Pamb_sea), SubS_9/2(Pamb_sea), SubS_8/2(Pamb_sea), SubS_7/2(Pamb_sea), SubS_6/2(Pamb_sea), SubS_5/2(Pamb_sea), SubS_4/2(Pamb_sea), SubS_3/2(Pamb_sea), SubS_2/2(Pamb_sea), SubS_1b/2(Pamb_sea)
  zero/1 -> >0/3
  >0/1 -> While_Iterator/3(IC)
  disp_clock/1 -> >0/1
  Half_time_1b/1 -> SubS_1b/4(HT)
  SubS_1b/1(bus) -> While_Iterator/23(In1b)

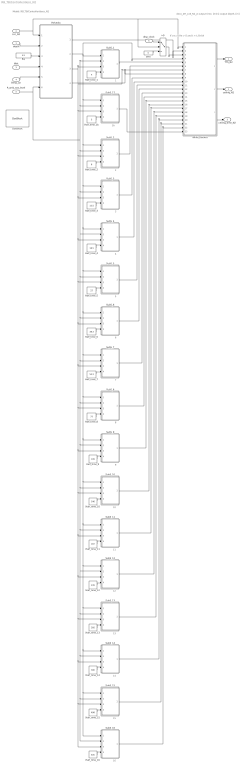
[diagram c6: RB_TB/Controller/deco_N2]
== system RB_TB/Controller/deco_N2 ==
  note: deco_ZH_L16_N2_w output time, [min]; output depth, [m]
  note: 1
  note: 2
  note: 3
  note: 4
  note: 5
  note: 6
  note: 7
  note: 8
  note: 9
  note: 10
  note: 11
  note: 12
  note: 13
  note: 14
  note: 15
  note: 16
  note: Model: RB_TB/Controller/deco_N2
  note: If cnc of He > 0 and t = t_finish
  note: 1b
  depth : Inport  Port=1  LatchInput=off
  cnc_N2 : Inport  Port=2  LatchInput=off
  Wet : Inport  Port=3  LatchInput=off
  Temp_air : Inport  Port=4  LatchInput=off
  P_amb_sea_level : Inport  Port=5  LatchInput=off
  disp_clock : Inport  Port=6  LatchInput=off
  >0 : Switch  Criteria=u2 > Threshold
  DocBlock : simulink/Model-Wide Utilities/DocBlock  DocumentType=Text
  Half_time_1 : Constant  Value=4
  Half_time_10 : Constant  Value=146
  Half_time_11 : Constant  Value=187
  Half_time_12 : Constant  Value=239
  Half_time_13 : Constant  Value=305
  Half_time_14 : Constant  Value=390
  Half_time_15 : Constant  Value=498
  Half_time_16 : Constant  Value=635
  Half_time_1b : Constant  Value=5
  Half_time_2 : Constant  Value=8
  Half_time_3 : Constant  Value=12.5
  Half_time_4 : Constant  Value=18.5
  Half_time_5 : Constant  Value=27
  Half_time_6 : Constant  Value=38.3
  Half_time_7 : Constant  Value=54.3
  Half_time_8 : Constant  Value=77
  Half_time_9 : Constant  Value=109
  Palveola : Subsystem
  RQ : Constant  Value=0.9
  SubS_1 : Subsystem
  SubS_10 : Subsystem
  SubS_11 : Subsystem
  SubS_12 : Subsystem
  SubS_13 : Subsystem
  SubS_14 : Subsystem
  SubS_15 : Subsystem
  SubS_16 : Subsystem
  SubS_17 : Subsystem
  SubS_2 : Subsystem
  SubS_3 : Subsystem
  SubS_4 : Subsystem
  SubS_5 : Subsystem
  SubS_6 : Subsystem
  SubS_7 : Subsystem
  SubS_8 : Subsystem
  SubS_9 : Subsystem
  While_Iterator : Subsystem  TreatAsAtomicUnit=on
  zero : Constant  Value=0
  TTS_N2 : Outport
  ceiling_N2 : Outport  Port=2
  ceiling_time_N2 : Outport  Port=3
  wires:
  P_amb_sea_level/1 -> Palveola/6(P_amb_see_level), SubS_15/2(Pamb_sea), SubS_16/2(Pamb_sea), SubS_14/2(Pamb_sea), SubS_13/2(Pamb_sea), SubS_12/2(Pamb_sea), SubS_11/2(Pamb_sea), SubS_10/2(Pamb_sea), SubS_9/2(Pamb_sea), SubS_8/2(Pamb_sea), SubS_7/2(Pamb_sea), SubS_6/2(Pamb_sea), SubS_5/2(Pamb_sea), SubS_4/2(Pamb_sea), SubS_3/2(Pamb_sea), SubS_2/2(Pamb_sea), SubS_1/2(Pamb_sea), SubS_17/2(Pamb_sea)
  Palveola/2(Palv) -> While_Iterator/4(Palv), SubS_1/1(Palv), SubS_15/1(Palv), SubS_16/1(Palv), SubS_14/1(Palv), SubS_13/1(Palv), SubS_12/1(Palv), SubS_11/1(Palv), SubS_10/1(Palv), SubS_9/1(Palv), SubS_8/1(Palv), SubS_7/1(Palv), SubS_6/1(Palv), SubS_5/1(Palv), SubS_4/1(Palv), SubS_3/1(Palv), SubS_2/1(Palv), SubS_17/1(Palv)
  Palveola/3(P_alv_INI) -> While_Iterator/7(Palv_INI), SubS_15/3(Palv_INI), SubS_16/3(Palv_INI), SubS_14/3(Palv_INI), SubS_13/3(Palv_INI), SubS_12/3(Palv_INI), SubS_11/3(Palv_INI), SubS_10/3(Palv_INI), SubS_9/3(Palv_INI), SubS_8/3(Palv_INI), SubS_7/3(Palv_INI), SubS_6/3(Palv_INI), SubS_5/3(Palv_INI), SubS_4/3(Palv_INI), SubS_3/3(Palv_INI), SubS_2/3(Palv_INI), SubS_17/3(Palv_INI), SubS_1/3(Palv_INI)
  depth/1 -> Palveola/2("depth, m ")
  cnc_N2/1 -> Palveola/1(Gas concentration), While_Iterator/1(cnc_N2), >0/2
  SubS_2/1(bus) -> While_Iterator/6(In2)
  SubS_1/1(bus) -> While_Iterator/5(In1)
  Palveola/1(Psw) -> While_Iterator/2(Psw)
  Palveola/4(fnc_hum_temp) -> While_Iterator/8(fnc_hum_temp)
  While_Iterator/1(TTS) -> TTS_N2/1
  While_Iterator/2(ceiling) -> ceiling_N2/1
  While_Iterator/3(ceiling_time) -> ceiling_time_N2/1
  RQ/1 -> Palveola/3(RQ)
  Wet/1 -> Palveola/4(Humidity)
  Temp_air/1 -> Palveola/5(Temperature)
  SubS_3/1(bus) -> While_Iterator/9(In3)
  SubS_4/1(bus) -> While_Iterator/10(In4)
  SubS_5/1(bus) -> While_Iterator/11(In5)
  SubS_6/1(bus) -> While_Iterator/12(In6)
  SubS_7/1(bus) -> While_Iterator/13(In7)
  SubS_8/1(bus) -> While_Iterator/14(In8)
  SubS_9/1(bus) -> While_Iterator/15(In9)
  SubS_10/1(bus) -> While_Iterator/16(In10)
  SubS_11/1(bus) -> While_Iterator/17(In11)
  SubS_12/1(bus) -> While_Iterator/18(In12)
  SubS_13/1(bus) -> While_Iterator/19(In13)
  SubS_14/1(bus) -> While_Iterator/20(In14)
  SubS_15/1(bus) -> While_Iterator/21(In15)
  SubS_16/1(bus) -> While_Iterator/22(In16)
  Half_time_1/1 -> SubS_1/4(HT)
  Half_time_2/1 -> SubS_2/4(HT)
  Half_time_3/1 -> SubS_3/4(HT)
  Half_time_4/1 -> SubS_4/4(HT)
  Half_time_5/1 -> SubS_5/4(HT)
  Half_time_6/1 -> SubS_6/4(HT)
  Half_time_7/1 -> SubS_7/4(HT)
  Half_time_8/1 -> SubS_8/4(HT)
  Half_time_9/1 -> SubS_9/4(HT)
  Half_time_10/1 -> SubS_10/4(HT)
  Half_time_11/1 -> SubS_11/4(HT)
  Half_time_12/1 -> SubS_12/4(HT)
  Half_time_13/1 -> SubS_13/4(HT)
  Half_time_14/1 -> SubS_14/4(HT)
  Half_time_15/1 -> SubS_15/4(HT)
  Half_time_16/1 -> SubS_16/4(HT)
  disp_clock/1 -> >0/1
  zero/1 -> >0/3
  >0/1 -> While_Iterator/3(IC)
  Half_time_1b/1 -> SubS_17/4(HT)
  SubS_17/1(bus) -> While_Iterator/23(In1b)

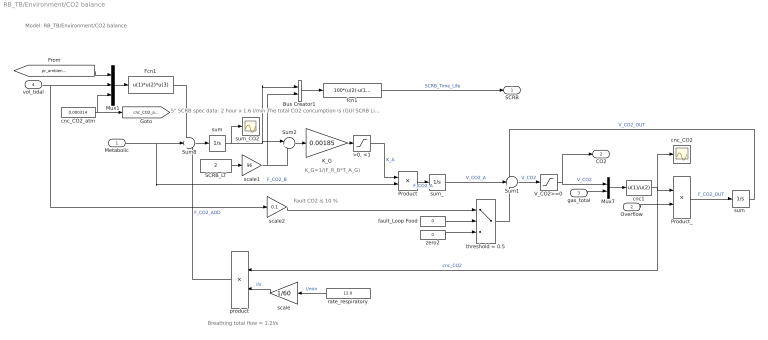
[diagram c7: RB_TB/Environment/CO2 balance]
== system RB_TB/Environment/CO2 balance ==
  note: Model: RB_TB/Environment/CO2 balance
  note: K_G=1/(F_R_B*T_A_G)
  note: Breathing total flow = 1.2l/s
  note: 5" SCRB spec data: 2 hour x 1.6 l/min The total CO2 concumption is (GUI SCRB Life-Time) x 192 / 2 litre
  note: Fault CO2 is 10 %
  Metabolic : Inport  Port=1  LatchInput=off
  Overflow : Inport  Port=2  LatchInput=off
  gas_total : Inport  Port=3  LatchInput=off
  vol_tidal : Inport  Port=4  LatchInput=off
  ">0, <1" : Saturate  UpperLimit=1  LowerLimit=0
  Bus Creator1 : BusCreator  DialogController=Simulink.DDGSource_Bus  Inputs=2
  Fcn1 : Fcn  Expr=u(1)*u(2)*u(3)
  K_G : Gain  Gain=0.00185
  Mux1 : Mux  Inputs=3
  Mux7 : Mux  Inputs=2
  Product : Product
  Product_ : Product
  SCRB_LT : Constant  Value=2
  Sum1 : Sum  Inputs=-++
  Sum2 : Sum  Inputs=|+-
  Sum8 : Sum  Inputs=+++
  V_CO2>=0 : Saturate  UpperLimit=inf  LowerLimit=0
  cnc1 : Fcn  Tag=ee  Priority=306454640  Expr=u(1)/u(2)
  cnc_CO2 : Scope
  cnc_CO2_atm : Constant  Value=0.000314
  fault_Loop Food : Constant  Value=0
  fcn1 : Fcn  Expr=100*(u(2)-u(1))/u(2)
  product : Product  Orientation=left
  rate_respiratory : Constant  Orientation=left  Value=12.0
  scale : Gain  Orientation=left  Gain=1/60
  scale1 : Gain  Gain=96
  scale2 : Gain  Gain=0.1
  sum : Integrator
  "sum " : Integrator
  sum_ : Integrator
  sum_CO2 : Scope
  threshold = 0.5 : Switch  Criteria=u2 > Threshold  Threshold=0.5
  zero2 : Constant  Value=0
  SCRB : Outport
  CO2 : Outport  Port=2
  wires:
  Metabolic/1 -> Product/2, Sum8/2  "F_CO2_B"
  Sum2/1 -> K_G/1
  K_G/1 -> ">0, <1"/1
  ">0, <1"/1 -> Product/1  "K_A"
  Product/1 -> sum_/1  "F_CO2_A"
  sum_/1 -> Sum1/2  "V_CO2_A"
  Sum1/1 -> V_CO2>=0/1  "V_CO2"
  Product_/1 -> "sum "/1  "F_CO2_OUT"
  "sum "/1 -> Sum1/1  "V_CO2_OUT"
  V_CO2>=0/1 -> Mux7/1, CO2/1  "V_CO2"
  Sum8/1 -> sum/1
  sum/1 -> Sum2/1, Bus Creator1/1, sum_CO2/1
  rate_respiratory/1 -> scale/1  "l/min"
  scale/1 -> product/2  "l/s"
  cnc_CO2_atm/1 -> [cnc_CO2_atm], Mux1/3
  vol_tidal/1 -> scale2/1, Mux1/2
  product/1 -> Sum8/3  "F_CO2_ADD"
  Fcn1/1 -> Sum8/1
  SCRB_LT/1 -> scale1/1
  Bus Creator1/1 -> fcn1/1
  fcn1/1 -> SCRB/1  "SCRB_Time_Life"
  scale1/1 -> Sum2/2, Bus Creator1/2
  threshold = 0.5/1 -> Sum1/3
  fault_Loop Food/1 -> threshold = 0.5/2
  scale2/1 -> threshold = 0.5/1
  zero2/1 -> threshold = 0.5/3
  Mux7/1 -> cnc1/1
  cnc1/1 -> cnc_CO2/1, Product_/1, product/1  "cnc_CO2"
  Overflow/1 -> Product_/2
  gas_total/1 -> Mux7/2
  [pr_ambient_sea_level] -> Mux1/1
  Mux1/1 -> Fcn1/1

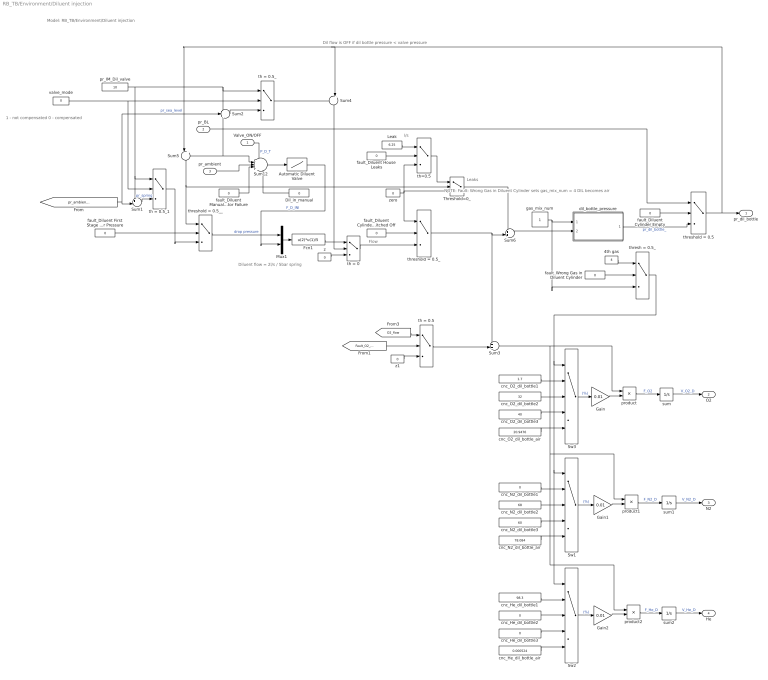
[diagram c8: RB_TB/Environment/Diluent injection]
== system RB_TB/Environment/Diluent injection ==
  note: Model: RB_TB/Environment/Diluent injection
  note: Diluent flow = 2l/s / 5bar spring
  note: NOTE: Fault: Wrong Gas in Diluent Cylinder sets gas_mix_num = 4 DIL becomes air
  note: Dil flow is OFF if dil bottle pressure < valve pressure
  note: 1 - not compensated 0 - compensated
  note: l/s
  note: Leaks
  note: Flow
  Valve_ON/OFF : Inport  Port=1  LatchInput=off
  pr_BL : Inport  Port=2  LatchInput=off
  pr_ambient : Inport  Port=3  LatchInput=off
  4th gas : Constant  Value=4
  Automatic Diluent Valve : Lookup  DialogController=Simulink.DDGSource  InputValues=[-10000 0.025 0.035 10000]  OutputValues=[0 0 1.2 1.2]  LookUpMeth=Interpolation-Use End Values
  Dil_in_manual : Constant  Orientation=left  Value=0
  Fcn1 : Fcn  Expr=u(2)*u(1)/5
  Gain : Gain  Gain=0.01
  Gain1 : Gain  Gain=0.01
  Gain2 : Gain  Gain=0.01
  Leak : Constant  Value=6.25
  Mux1 : Mux  Inputs=2
  Sum1 : Sum  Inputs=+-|
  Sum12 : Sum  Inputs=+-+++
  Sum2 : Sum  Inputs=+-+
  Sum3 : Sum  Inputs=++|
  Sum4 : Sum  Orientation=down  Inputs=-+|
  Sum5 : Sum  Orientation=down  Inputs=|+-
  Sum6 : Sum  Inputs=++|
  Sw1 : MultiPortSwitch
  Sw2 : MultiPortSwitch
  Sw3 : MultiPortSwitch
  Threshold=0_ : Switch  Criteria=u2 > Threshold
  cnc_He_dil_bottle1 : Constant  Value=98.3
  cnc_He_dil_bottle2 : Constant  Value=0
  cnc_He_dil_bottle3 : Constant  Value=0
  cnc_He_dil_bottle_air : Constant  Value=0.000524
  cnc_N2_dil_bottle1 : Constant  Value=0
  cnc_N2_dil_bottle2 : Constant  Value=68
  cnc_N2_dil_bottle3 : Constant  Value=60
  cnc_N2_dil_bottle_air : Constant  Value=78.084
  cnc_O2_dil_bottle1 : Constant  Value=1.7
  cnc_O2_dil_bottle2 : Constant  Value=32
  cnc_O2_dil_bottle3 : Constant  Value=40
  cnc_O2_dil_bottle_air : Constant  Value=20.9476
  dil_bottle_pressure : Subsystem
  fault_Diluent Cylinder Empty : Constant  Value=0
  fault_Diluent Cylinder Switched Off : Constant  Value=0
  fault_Diluent First Stage Over Pressure : Constant  Value=0
  fault_Diluent House Leaks : Constant  Value=0
  fault_Diluent Manual Injector Failure : Constant  Value=0
  fault_Wrong Gas in Diluent Cylinder : Constant  Value=0
  gas_mix_num : Constant
  pr_IM_Dil_valve : Constant  Value=10
  product : Product
  product1 : Product
  product2 : Product
  sum : Integrator
  sum1 : Integrator
  sum2 : Integrator
  th = 0 : Switch  Criteria=u2 > Threshold
  th = 0.5 : Switch  Criteria=u2 > Threshold  Threshold=0.5
  th = 0.5_ : Switch  Criteria=u2 > Threshold
  th = 0.5_1 : Switch  Criteria=u2 > Threshold
  th=0.5 : Switch  Criteria=u2 > Threshold  Threshold=0.5
  thresh = 0.5_ : Switch  Criteria=u2 > Threshold  Threshold=0.5
  threshold = 0.5 : Switch  Criteria=u2 > Threshold  Threshold=0.5
  threshold = 0.5_ : Switch  Criteria=u2 > Threshold  Threshold=0.5
  threshold = 0.5__ : Switch  Criteria=u2 > Threshold  Threshold=0.5
  valve_mode : Constant  Value=0
  z : Constant  Value=0
  z1 : Constant  Value=0
  zero : Constant  Value=0
  pr_dil_bottle : Outport
  O2 : Outport  Port=2
  N2 : Outport  Port=3
  He : Outport  Port=4
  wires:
  zero/1 -> Threshold=0_/3, th=0.5/3, threshold = 0.5_/1
  gas_mix_num/1 -> dil_bottle_pressure/1(gas_mix), thresh = 0.5_/3
  product/1 -> sum/1  "F_O2"
  sum/1 -> O2/1  "V_O2_D"
  sum1/1 -> N2/1  "V_N2_D"
  product1/1 -> sum1/1  "F_N2_D"
  sum2/1 -> He/1  "V_He_D"
  product2/1 -> sum2/1  "F_He_D"
  cnc_He_dil_bottle3/1 -> Sw2/4
  cnc_N2_dil_bottle2/1 -> Sw1/3
  cnc_O2_dil_bottle1/1 -> Sw3/2
  Sw3/1 -> Gain/1  "(%)"
  Gain/1 -> product/2
  Gain1/1 -> product1/2
  Gain2/1 -> product2/2
  Sw2/1 -> Gain2/1  "(%)"
  dil_bottle_pressure/1(O2) -> threshold = 0.5/3  "pr_dil_bottle_"
  cnc_O2_dil_bottle2/1 -> Sw3/3
  cnc_O2_dil_bottle3/1 -> Sw3/4
  cnc_N2_dil_bottle1/1 -> Sw1/2
  cnc_N2_dil_bottle3/1 -> Sw1/4
  cnc_He_dil_bottle1/1 -> Sw2/2
  cnc_He_dil_bottle2/1 -> Sw2/3
  threshold = 0.5/1 -> pr_dil_bottle/1, Sum5/1, Sum4/2
  fault_Diluent Cylinder Empty/1 -> threshold = 0.5/2
  z/1 -> th = 0/3
  pr_BL/1 -> Sum2/3, Sum12/2, Sum5/2, threshold = 0.5/1
  fault_Diluent Cylinder Switched Off/1 -> threshold = 0.5_/2
  th = 0/1 -> threshold = 0.5_/3
  threshold = 0.5_/1 -> Sum6/2, Sum3/1
  Sw1/1 -> Gain1/1  "(%)"
  cnc_O2_dil_bottle_air/1 -> Sw3/5
  cnc_N2_dil_bottle_air/1 -> Sw1/5
  cnc_He_dil_bottle_air/1 -> Sw2/5
  [O2_flow] -> th = 0.5/1
  [Fault_O2_wrong] -> th = 0.5/2
  z1/1 -> th = 0.5/3
  th = 0.5/1 -> Sum3/2
  Sum3/1 -> product1/1, product2/1, product/1
  valve_mode/1 -> th = 0.5_/2, th = 0.5_1/2
  Sum2/1 -> th = 0.5_/3
  Sum4/1 -> th = 0/2
  Automatic Diluent Valve/1 -> Mux1/2  "F_D_INI"
  Mux1/1 -> Fcn1/1
  Fcn1/1 -> th = 0/1
  fault_Diluent First Stage Over Pressure/1 -> threshold = 0.5__/2
  threshold = 0.5__/1 -> Mux1/1  "drop pressure"
  Sum5/1 -> threshold = 0.5__/1, Threshold=0_/2
  fault_Diluent House Leaks/1 -> th=0.5/2
  Leak/1 -> th=0.5/1
  Sum6/1 -> dil_bottle_pressure/2(F_D)
  Threshold=0_/1 -> Sum6/1
  th=0.5/1 -> Threshold=0_/1
  pr_IM_Dil_valve/1 -> th = 0.5_/1, Sum2/1, th = 0.5_1/1, Sum1/1
  th = 0.5_/1 -> Sum4/1
  th = 0.5_1/1 -> threshold = 0.5__/3
  [pr_ambient_sea_level] -> Sum1/2, Sum2/2  "pr_sea_level"
  Sum1/1 -> th = 0.5_1/3  "pr_spring"
  fault_Wrong Gas in Diluent Cylinder/1 -> thresh = 0.5_/2
  4th gas/1 -> thresh = 0.5_/1
  thresh = 0.5_/1 -> Sw3/1, Sw1/1, Sw2/1
  Sum12/1 -> Automatic Diluent Valve/1
  pr_ambient/1 -> Sum12/3
  Valve_ON/OFF/1 -> Sum12/1  "P_D_T"
  fault_Diluent Manual Injector Failure/1 -> Sum12/4
  Dil_in_manual/1 -> Sum12/5

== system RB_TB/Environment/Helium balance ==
  note: V_He_BL_ini
  note: Model: RB_TB/Environment/Helium balance
  V_He_dil : Inport  Port=1  LatchInput=off
  gas_total : Inport  Port=2  LatchInput=off
  Overflow : Inport  Port=3  LatchInput=off
  vol_tidal : Inport  Port=4  LatchInput=off
  Fcn1 : Fcn  Expr=u(1)*u(2)*u(3)
  Mux1 : Mux  Inputs=3
  Mux3 : Mux  Inputs=2
  Product_ : Product
  Sum5 : Sum  Inputs=++-
  V_He>=0 : Saturate  UpperLimit=inf  LowerLimit=0
  cnc3 : Fcn  Tag=ee  Priority=306454640  Expr=u(1)/u(2)
  cnc_He : Scope
  sum : Integrator
  He inside : Outport
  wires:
  V_He_dil/1 -> Sum5/2  "V_He_D"
  Fcn1/1 -> Sum5/1
  V_He>=0/1 -> He inside/1, Mux3/1  "V_He"
  Sum5/1 -> V_He>=0/1  "V_He"
  sum/1 -> Sum5/3  "V_He_OUT"
  Product_/1 -> sum/1  "F_He_OUT"
  Mux3/1 -> cnc3/1
  cnc3/1 -> [cnc_He_presize], cnc_He/1, Product_/1
  gas_total/1 -> Mux3/2
  Overflow/1 -> Product_/2
  vol_tidal/1 -> Mux1/2
  [pr_ambient_sea_level] -> Mux1/1
  Mux1/1 -> Fcn1/1
  [cnc_He_atm] -> Mux1/3

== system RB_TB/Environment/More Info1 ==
  note: NOTE:
  note: This subsystem models a breathing loop gas changing.
  note: Block: RB_TB/Environment/More Info
